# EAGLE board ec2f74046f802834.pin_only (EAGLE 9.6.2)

Size 55.88 x 58.42 mm. Coordinates in mm from the lower left corner, seen from the top.
Outline: 0,55.88 0,2.54 arc90 2.54,0 53.34,0 arc90 55.88,2.54 55.88,55.88 arc90 53.34,58.42 2.54,58.42 arc90 0,55.88
Copper layers (1*16): Top 0.035mm / dielectric 1.5mm / Bottom 0.035mm
Design rules "default *": minimum track width 8mil, minimum drill 24mil, track to track 9mil, track to pad 8mil, pad to pad 8mil, via to via 8mil, smd to smd 8mil, copper to edge 10mil, drill to drill 8mil, minimum pad ring 10mil, minimum via ring 8mil, stop-mask expansion 4mil, vias tented up to drill 0mil, thermal gap 10mil

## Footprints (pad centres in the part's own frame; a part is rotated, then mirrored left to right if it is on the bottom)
1X40-0.5MM = smd 0.25 x 2: 1 -9.75,0; 2 -9.25,0; 3 -8.75,0; 4 -8.25,0; 5 -7.75,0; 6 -7.25,0; 7 -6.75,0; 8 -6.25,0; 9 -5.75,0; 10 -5.25,0; 11 -4.75,0; 12 -4.25,0; 13 -3.75,0; 14 -3.25,0; 15 -2.75,0; 16 -2.25,0; 17 -1.75,0; 18 -1.25,0; 19 -0.75,0; 20 -0.25,0; 21 0.25,0; 22 0.75,0; 23 1.25,0; 24 1.75,0; 25 2.25,0; 26 2.75,0; 27 3.25,0; 28 3.75,0; 29 4.25,0; 30 4.75,0; 31 5.25,0; 32 5.75,0; 33 6.25,0; 34 6.75,0; 35 7.25,0; 36 7.75,0; 37 8.25,0; 38 8.75,0; 39 9.25,0; 40 9.75,0
2X20-BIG = drill 1.016 pad 1.778 octagon: 1 -24.13,-1.27; 2 -24.13,1.27; 3 -21.59,-1.27; 4 -21.59,1.27; 5 -19.05,-1.27; 6 -19.05,1.27; 7 -16.51,-1.27; 8 -16.51,1.27; 9 -13.97,-1.27; 10 -13.97,1.27; 11 -11.43,-1.27; 12 -11.43,1.27; 13 -8.89,-1.27; 14 -8.89,1.27; 15 -6.35,-1.27; 16 -6.35,1.27; 17 -3.81,-1.27; 18 -3.81,1.27; 19 -1.27,-1.27; 20 -1.27,1.27; 21 1.27,-1.27; 22 1.27,1.27; 23 3.81,-1.27; 24 3.81,1.27; 25 6.35,-1.27; 26 6.35,1.27; 27 8.89,-1.27; 28 8.89,1.27; 29 11.43,-1.27; 30 11.43,1.27; 31 13.97,-1.27; 32 13.97,1.27; 33 16.51,-1.27; 34 16.51,1.27; 35 19.05,-1.27; 36 19.05,1.27; 37 21.59,-1.27; 38 21.59,1.27; 39 24.13,-1.27; 40 24.13,1.27
1X20-BIG = drill 1.016 pad 1.778: 1 -24.13,0; 2 -21.59,0; 3 -19.05,0; 4 -16.51,0; 5 -13.97,0; 6 -11.43,0; 7 -8.89,0; 8 -6.35,0; 9 -3.81,0; 10 -1.27,0; 11 1.27,0; 12 3.81,0; 13 6.35,0; 14 8.89,0; 15 11.43,0; 16 13.97,0; 17 16.51,0; 18 19.05,0; 19 21.59,0; 20 24.13,0
1X40-0.6MM = smd 0.3 x 1.6: 1 -11.7,0; 2 -11.1,0; 3 -10.5,0; 4 -9.9,0; 5 -9.3,0; 6 -8.7,0; 7 -8.1,0; 8 -7.5,0; 9 -6.9,0; 10 -6.3,0; 11 -5.7,0; 12 -5.1,0; 13 -4.5,0; 14 -3.9,0; 15 -3.3,0; 16 -2.7,0; 17 -2.1,0; 18 -1.5,0; 19 -0.9,0; 20 -0.3,0; 21 0.3,0; 22 0.9,0; 23 1.5,0; 24 2.1,0; 25 2.7,0; 26 3.3,0; 27 3.9,0; 28 4.5,0; 29 5.1,0; 30 5.7,0; 31 6.3,0; 32 6.9,0; 33 7.5,0; 34 8.1,0; 35 8.7,0; 36 9.3,0; 37 9.9,0; 38 10.5,0; 39 11.1,0; 40 11.7,0
1X40-0.7MM = smd 0.35 x 1.6: 1 -13.65,0; 2 -12.95,0; 3 -12.25,0; 4 -11.55,0; 5 -10.85,0; 6 -10.15,0; 7 -9.45,0; 8 -8.75,0; 9 -8.05,0; 10 -7.35,0; 11 -6.65,0; 12 -5.95,0; 13 -5.25,0; 14 -4.55,0; 15 -3.85,0; 16 -3.15,0; 17 -2.45,0; 18 -1.75,0; 19 -1.05,0; 20 -0.35,0; 21 0.35,0; 22 1.05,0; 23 1.75,0; 24 2.45,0; 25 3.15,0; 26 3.85,0; 27 4.55,0; 28 5.25,0; 29 5.95,0; 30 6.65,0; 31 7.35,0; 32 8.05,0; 33 8.75,0; 34 9.45,0; 35 10.15,0; 36 10.85,0; 37 11.55,0; 38 12.25,0; 39 12.95,0; 40 13.65,0
1X40-0.8MM = smd 0.4 x 2: 1 -15.6,0; 2 -14.8,0; 3 -14,0; 4 -13.2,0; 5 -12.4,0; 6 -11.6,0; 7 -10.8,0; 8 -10,0; 9 -9.2,0; 10 -8.4,0; 11 -7.6,0; 12 -6.8,0; 13 -6,0; 14 -5.2,0; 15 -4.4,0; 16 -3.6,0; 17 -2.8,0; 18 -2,0; 19 -1.2,0; 20 -0.4,0; 21 0.4,0; 22 1.2,0; 23 2,0; 24 2.8,0; 25 3.6,0; 26 4.4,0; 27 5.2,0; 28 6,0; 29 6.8,0; 30 7.6,0; 31 8.4,0; 32 9.2,0; 33 10,0; 34 10.8,0; 35 11.6,0; 36 12.4,0; 37 13.2,0; 38 14,0; 39 14.8,0; 40 15.6,0
1X40-1MM = smd 0.5 x 3: 1 -19.5,-0.17; 2 -18.5,-0.17; 3 -17.5,-0.17; 4 -16.5,-0.17; 5 -15.5,-0.17; 6 -14.5,-0.17; 7 -13.5,-0.17; 8 -12.5,-0.17; 9 -11.5,-0.17; 10 -10.5,-0.17; 11 -9.5,-0.17; 12 -8.5,-0.17; 13 -7.5,-0.17; 14 -6.5,-0.17; 15 -5.5,-0.17; 16 -4.5,-0.17; 17 -3.5,-0.17; 18 -2.5,-0.17; 19 -1.5,-0.17; 20 -0.5,-0.17; 21 0.5,-0.17; 22 1.5,-0.17; 23 2.5,-0.17; 24 3.5,-0.17; 25 4.5,-0.17; 26 5.5,-0.17; 27 6.5,-0.17; 28 7.5,-0.17; 29 8.5,-0.17; 30 9.5,-0.17; 31 10.5,-0.17; 32 11.5,-0.17; 33 12.5,-0.17; 34 13.5,-0.17; 35 14.5,-0.17; 36 15.5,-0.17; 37 16.5,-0.17; 38 17.5,-0.17; 39 18.5,-0.17; 40 19.5,-0.17

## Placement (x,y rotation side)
CON1  PINHD-1X40-0.5MM  [1X40-0.5MM]  27.94,30.8 0 top
JP1  [2X20-BIG]  27.94,2.54 0 top
JP2  [1X20-BIG]  1.27,31.75 90 top
JP3  [1X20-BIG]  54.61,31.75 270 top
U$1  PINHD-1X40-0.6MM  [1X40-0.6MM]  27.94,24.89 0 top
U$2  PINHD-1X40-0.7MM  [1X40-0.7MM]  27.94,20.32 0 top
U$3  PINHD-1X40-0.8MM  [1X40-0.8MM]  27.94,16.51 0 top
U$4  PINHD-1X40-1MM  [1X40-1MM]  27.94,11.43 0 top
U$5  [ADAFRUIT_TEXT_20MM]  16.13,47.55 0 top

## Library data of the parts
CON1 JP1-JP3 U$1-U$4 = adafruit
U$5 = microbuilder

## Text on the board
tPlace: 20 | 21 | 19 | 22 | 18 | 23 | 17 | 24 | 16 | 25 | 15 | 26 | Ladyada's Super Lucky / 40-Pin FPC to Breadboard / Adapter Plate! | 14 | 27 | 13 | 28 | 12 | 0.5mm/0.6mm/0.7mm/0.8mm/1.0mm | 29 | 11 | 0.5mm | 30 | 10 | 31 | 9 | 32 | 0.6mm | 8 | 33 | 7 | 34 | 0.7mm | 6 | 35 | 5 | 0.8mm | 36 | 4 | 37 | 3 | 1mm | 38 | 2 | 39 | 1 | 40 | 2 | 4 | 6 | 8 | 10 | 12 | 14 | 16 | 18 | 20 | 22 | 24 | 26 | 28 | 30 | 32 | 34 | 36 | 38

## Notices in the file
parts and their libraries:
microbuilder: This work is placed in the public domain, and may be freely used for commercial and non-commercial work with the following conditions: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
